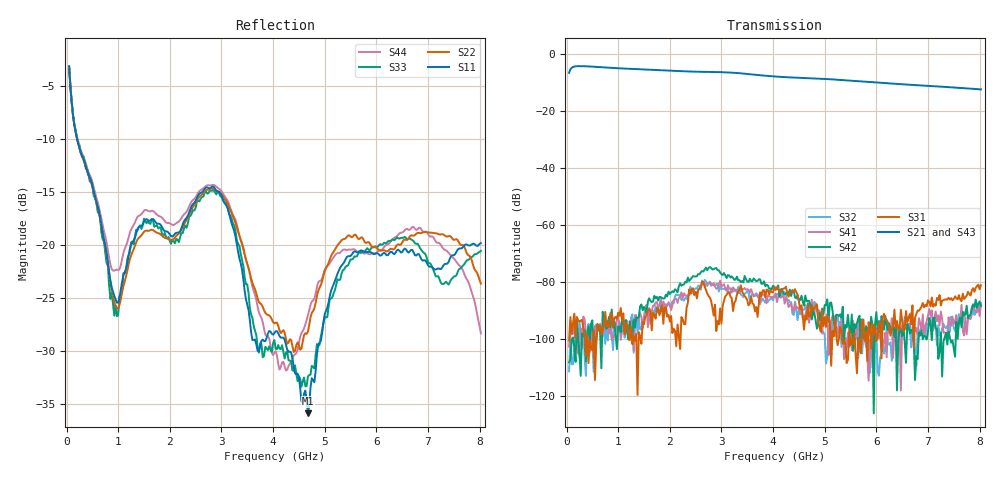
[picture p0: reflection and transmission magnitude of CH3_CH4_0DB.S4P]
! "!Agilent Technologies,E5071C,MY46316741,A.11.02"
!Date: Thu May 28 15:05:39 2026
!Data & Calibration Information:
!1:CH3 INPUT 2:CH3 OUTPUT 3:CH4 INPUT 4:CH4 OUTPUT
!Freq	S11:SOLT4(ON)	S12:SOLT4(ON)	S13:SOLT4(ON)	S14:SOLT4(ON)
!	S21:SOLT4(ON)	S22:SOLT4(ON)	S23:SOLT4(ON)	S24:SOLT4(ON)
!	S31:SOLT4(ON)	S32:SOLT4(ON)	S33:SOLT4(ON)	S34:SOLT4(ON)
!	S41:SOLT4(ON)	S42:SOLT4(ON)	S43:SOLT4(ON)	S44:SOLT4(ON)
!PortZ  Port1:50+j0  Port2:50+j0  Port3:50+j0  Port4:50+j0
!Above PortZ is port z conversion or system Z0 setting when saving the data.
! "!When reading, reference impedance value at option line is always used."
# Hz S dB R 50
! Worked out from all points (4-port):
!   320 points, 50 MHz to 8.025 GHz, reference 50 ohm
!   strongest paths, dB at 50 MHz, 2.05 GHz, 4.05 GHz, 6.05 GHz, 8.025 GHz:
!     S21: -6.5, -5.8, -7.8, -10.0, -12.3
!     S43: -6.5, -5.8, -7.9, -10.1, -12.5
!     S31: -100.5, -97.9, -82.8, -95.1, -81.1
!     S42: -108.2, -83.3, -82.6, -93.7, -88.4
!     S41: -102.7, -88.1, -84.0, -99.9, -88.1
!     S32: -111.4, -86.8, -85.2, -113.0, -87.4
!   lowest |S11| = -35.9 dB at 4.675 GHz (marker M1), VSWR 1.03, Z = 49 - j1.26 ohm
!   |S11| at or under -10 dB: 206.1 MHz to end of sweep
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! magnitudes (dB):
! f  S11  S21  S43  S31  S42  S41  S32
! 50 MHz  -3.2  -6.5  -6.5  -100.5  -108.2  -102.7  -111.4
! 925 MHz  -24.8  -4.8  -4.9  -92.5  -93.8  -99.4  -94.5
! 2.85 GHz  -14.5  -6.2  -6.3  -91.8  -75.5  -80.4  -81.0
! 4.125 GHz  -28.6  -7.9  -8.0  -83.2  -85.2  -83.9  -84.9
! 4.675 GHz  -35.9  -8.4  -8.5  -87.5  -86.6  -92.2  -87.5
! 5.425 GHz  -21.2  -9.2  -9.2  -108.5  -96.0  -103.0  -100.2
! 8.025 GHz  -19.8  -12.3  -12.5  -81.1  -88.4  -88.1  -87.4
